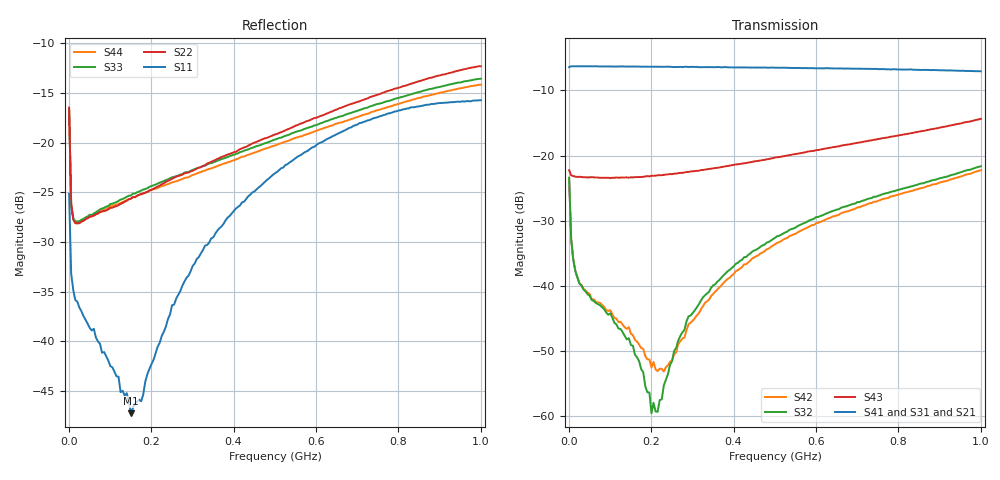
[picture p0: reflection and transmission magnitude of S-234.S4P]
!Agilent Technologies,E5071B,MY42300999,A.09.10
!Date: Thu Apr 13 17:02:36 2023
!Data & Calibration Information:
!Freq	S11:SOLT4(ON)	S12:SOLT4(ON)	S13:SOLT4(ON)	S14:SOLT4(ON)
!	S21:SOLT4(ON)	S22:SOLT4(ON)	S23:SOLT4(ON)	S24:SOLT4(ON)
!	S31:SOLT4(ON)	S32:SOLT4(ON)	S33:SOLT4(ON)	S34:SOLT4(ON)
!	S41:SOLT4(ON)	S42:SOLT4(ON)	S43:SOLT4(ON)	S44:SOLT4(ON)
# Hz S RI R 50
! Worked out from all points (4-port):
!   201 points, 1 MHz to 1 GHz, reference 50 ohm
!   strongest paths, dB at 1 MHz, 250.8 MHz, 500.5 MHz, 750.2 MHz, 1 GHz:
!     S41: -6.4, -6.4, -6.5, -6.7, -7.1
!     S31: -6.4, -6.4, -6.5, -6.8, -7.1
!     S21: -6.4, -6.4, -6.6, -6.9, -7.2
!     S43: -22.3, -22.9, -20.3, -17.5, -14.4
!     S32: -23.4, -51.6, -32.6, -26.2, -21.6
!     S42: -23.4, -51.5, -33.6, -27.0, -22.3
!   lowest |S11| = -47.2 dB at 150.8 MHz (marker M1), VSWR 1.01, Z = 50.1 + j0.421 ohm
!   |S11| at or under -10 dB: start of sweep to end of sweep
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1000000  -0.0347 0.0432  0.4765 0.0194  0.4778 0.0192  0.478 0.0192
         0.4771 0.0195  -0.0628 0.1365  0.0507 -0.0447  0.0508 -0.0447
         0.4777 0.0199  0.0507 -0.0446  -0.0608 0.134  -0.0773 -0.000364
         0.4778 0.0198  0.0507 -0.0445  -0.0772 -0.000425  -0.0603 0.1337
5995000  -0.0179 0.0127  0.4844 -0.00394  0.4849 -0.00376  0.486 -0.0036
         0.485 -0.00397  0.0194 0.0451  0.0147 -0.0175  0.0147 -0.0175
         0.4853 -0.00451  0.0147 -0.0174  0.0207 0.0445  -0.0706 0.00393
         0.4852 -0.00402  0.0146 -0.0174  -0.0704 0.0039  0.0209 0.0441
2.5975e7  -0.0126 0.00766  0.4826 -0.0384  0.484 -0.0389  0.4843 -0.0378
          0.4837 -0.038  0.0357 0.0165  0.00817 -0.00644  0.00807 -0.00658
          0.485 -0.0382  0.0081 -0.00649  0.0364 0.0174  -0.0683 0.00791
          0.4847 -0.0384  0.00807 -0.00666  -0.0683 0.00801  0.0364 0.0163
1.5085e8  0.00111 0.0042  0.4303 -0.2164  0.4298 -0.2173  0.4306 -0.2143
          0.4284 -0.2168  0.0522 -0.0027  0.00187 -0.00303  0.00167 -0.00395
          0.4317 -0.217  0.0019 -0.00295  0.0542 0.000835  -0.06 0.0318
          0.4328 -0.2137  0.00166 -0.00395  -0.0601 0.0319  0.0519 -0.0045
2.008e8  0.00765 0.000719  0.3885 -0.2796  0.392 -0.2797  0.394 -0.2757
         0.3893 -0.279  0.0571 -0.0101  -0.000331 -0.00095  -0.000599 -0.00224
         0.3911 -0.2799  -0.000421 -0.000957  0.0602 -0.00546  -0.0564 0.0407
         0.3933 -0.2774  -0.000685 -0.00225  -0.0566 0.041  0.0565 -0.0121
4.05595e8  0.0198 -0.0422  0.1413 -0.4484  0.1437 -0.4532  0.1504 -0.4509
           0.141 -0.4494  0.0701 -0.0564  -0.00464 0.0141  -0.00582 0.0116
           0.1427 -0.4522  -0.00472 0.014  0.0739 -0.0473  -0.0368 0.0769
           0.15 -0.4525  -0.00585 0.0116  -0.0368 0.0772  0.062 -0.054
1e9  -0.1075 0.1232  -0.4053 0.1545  -0.4121 0.1533  -0.4223 0.1344
     -0.4069 0.1545  -0.1388 -0.1985  0.0704 0.0443  0.0659 0.0408
     -0.4116 0.1535  0.0701 0.044  -0.1097 -0.1789  0.1245 0.1452
     -0.423 0.1347  0.0656 0.0405  0.1246 0.1454  -0.0995 -0.1685
